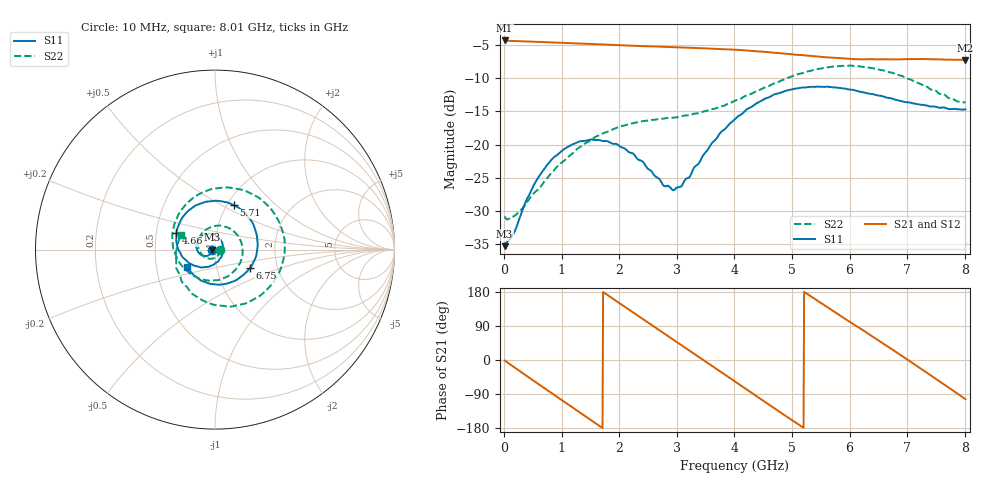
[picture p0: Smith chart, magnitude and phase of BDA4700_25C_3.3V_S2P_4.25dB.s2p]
!Agilent Technologies,E5071B,MY42404982,A.09.10
!Date: Mon Oct 20 18:04:46 2025
!Data & Calibration Information:
!Freq	S11:SOLT2(ON)	S21:SOLT2(ON)	S12:SOLT2(ON)	S22:SOLT2(ON)
# Hz S RI R 50
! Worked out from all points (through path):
!   801 points, 10 MHz to 8.01 GHz, reference 50 ohm
!   highest |S21| = -4.37 dB at 10 MHz (marker M1); lowest = -7.3 dB at 8.01 GHz (marker M2)
!   group delay of S21, straight-line fit = 284 ps
!   lowest |S11| = -35.3 dB at 10 MHz (marker M3), VSWR 1.04, Z = 48.3 - j0.121 ohm
!   |S11| at or under -10 dB: start of sweep to end of sweep
!   |S22| runs from -31.3 to -8.1 dB; largest |S21 - S12| = 0.0071
!   S11 on the Smith chart (normalised r, x): 10 MHz: 0.97, -0.00; 4.66 GHz: 0.64, +0.13; 5.71 GHz: 1.07, +0.57; 6.75 GHz: 1.44, -0.32; 8.01 GHz: 0.72, -0.15
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1e7  -0.0172 -0.00125  0.6045 -0.013  0.6044 -0.0134  0.0288 -0.00254
3.3e8  -0.0242 -0.0225  0.4857 -0.3442  0.4857 -0.3443  0.0207 -0.0263
7.2e8  -0.0572 -0.036  0.1382 -0.5704  0.1384 -0.5703  -0.0181 -0.051
1.02e9  -0.0885 -0.0203  -0.177 -0.5525  -0.177 -0.5527  -0.0647 -0.0364
1.35e9  -0.1043 0.0196  -0.4523 -0.3512  -0.4524 -0.3512  -0.0941 0.0262
1.93e9  -0.0553 0.0847  -0.5166 0.2129  -0.5166 0.2132  0.0028 0.1319
2.32e9  0.00229 0.0776  -0.2535 0.4882  -0.2532 0.488  0.1135 0.0937
2.68e9  0.0404 0.0384  0.0907 0.5361  0.0898 0.5354  0.154 -0.0188
2.96e9  0.0449 -0.00832  0.3337 0.4219  0.333 0.421  0.1179 -0.1072
3.37e9  0.00963 -0.0707  0.5227 0.087  0.5232 0.0866  -0.00686 -0.1711
4.01e9  -0.132 -0.0817  0.2821 -0.431  0.2828 -0.4299  -0.2024 -0.0658
4.33e9  -0.1956 -0.0149  0.002 -0.5035  0.00135 -0.5044  -0.2379 0.0587
4.66e9  -0.2146 0.0931  -0.2741 -0.4063  -0.2733 -0.4076  -0.2003 0.2013
5.01e9  -0.159 0.2062  -0.4456 -0.1649  -0.4467 -0.1655  -0.0675 0.3193
5.35e9  -0.0411 0.2679  -0.4473 0.1138  -0.4478 0.1114  0.1207 0.3388
5.71e9  0.1046 0.2477  -0.2874 0.3446  -0.2868 0.3445  0.3065 0.2323
6.18e9  0.2258 0.1056  0.0489 0.4338  0.0537 0.4343  0.3826 -0.0465
6.68e9  0.2081 -0.0828  0.3629 0.2416  0.3639 0.2409  0.2056 -0.283
6.75e9  0.1944 -0.1042  0.389 0.1962  0.3907 0.1932  0.1687 -0.3007
7.29e9  0.0327 -0.1953  0.3858 -0.2082  0.3854 -0.2092  -0.1202 -0.2511
7.66e9  -0.0809 -0.1703  0.1718 -0.3989  0.171 -0.3998  -0.2178 -0.0888
8.01e9  -0.155 -0.0987  -0.0998 -0.4196  -0.0984 -0.42  -0.1897 0.0812
